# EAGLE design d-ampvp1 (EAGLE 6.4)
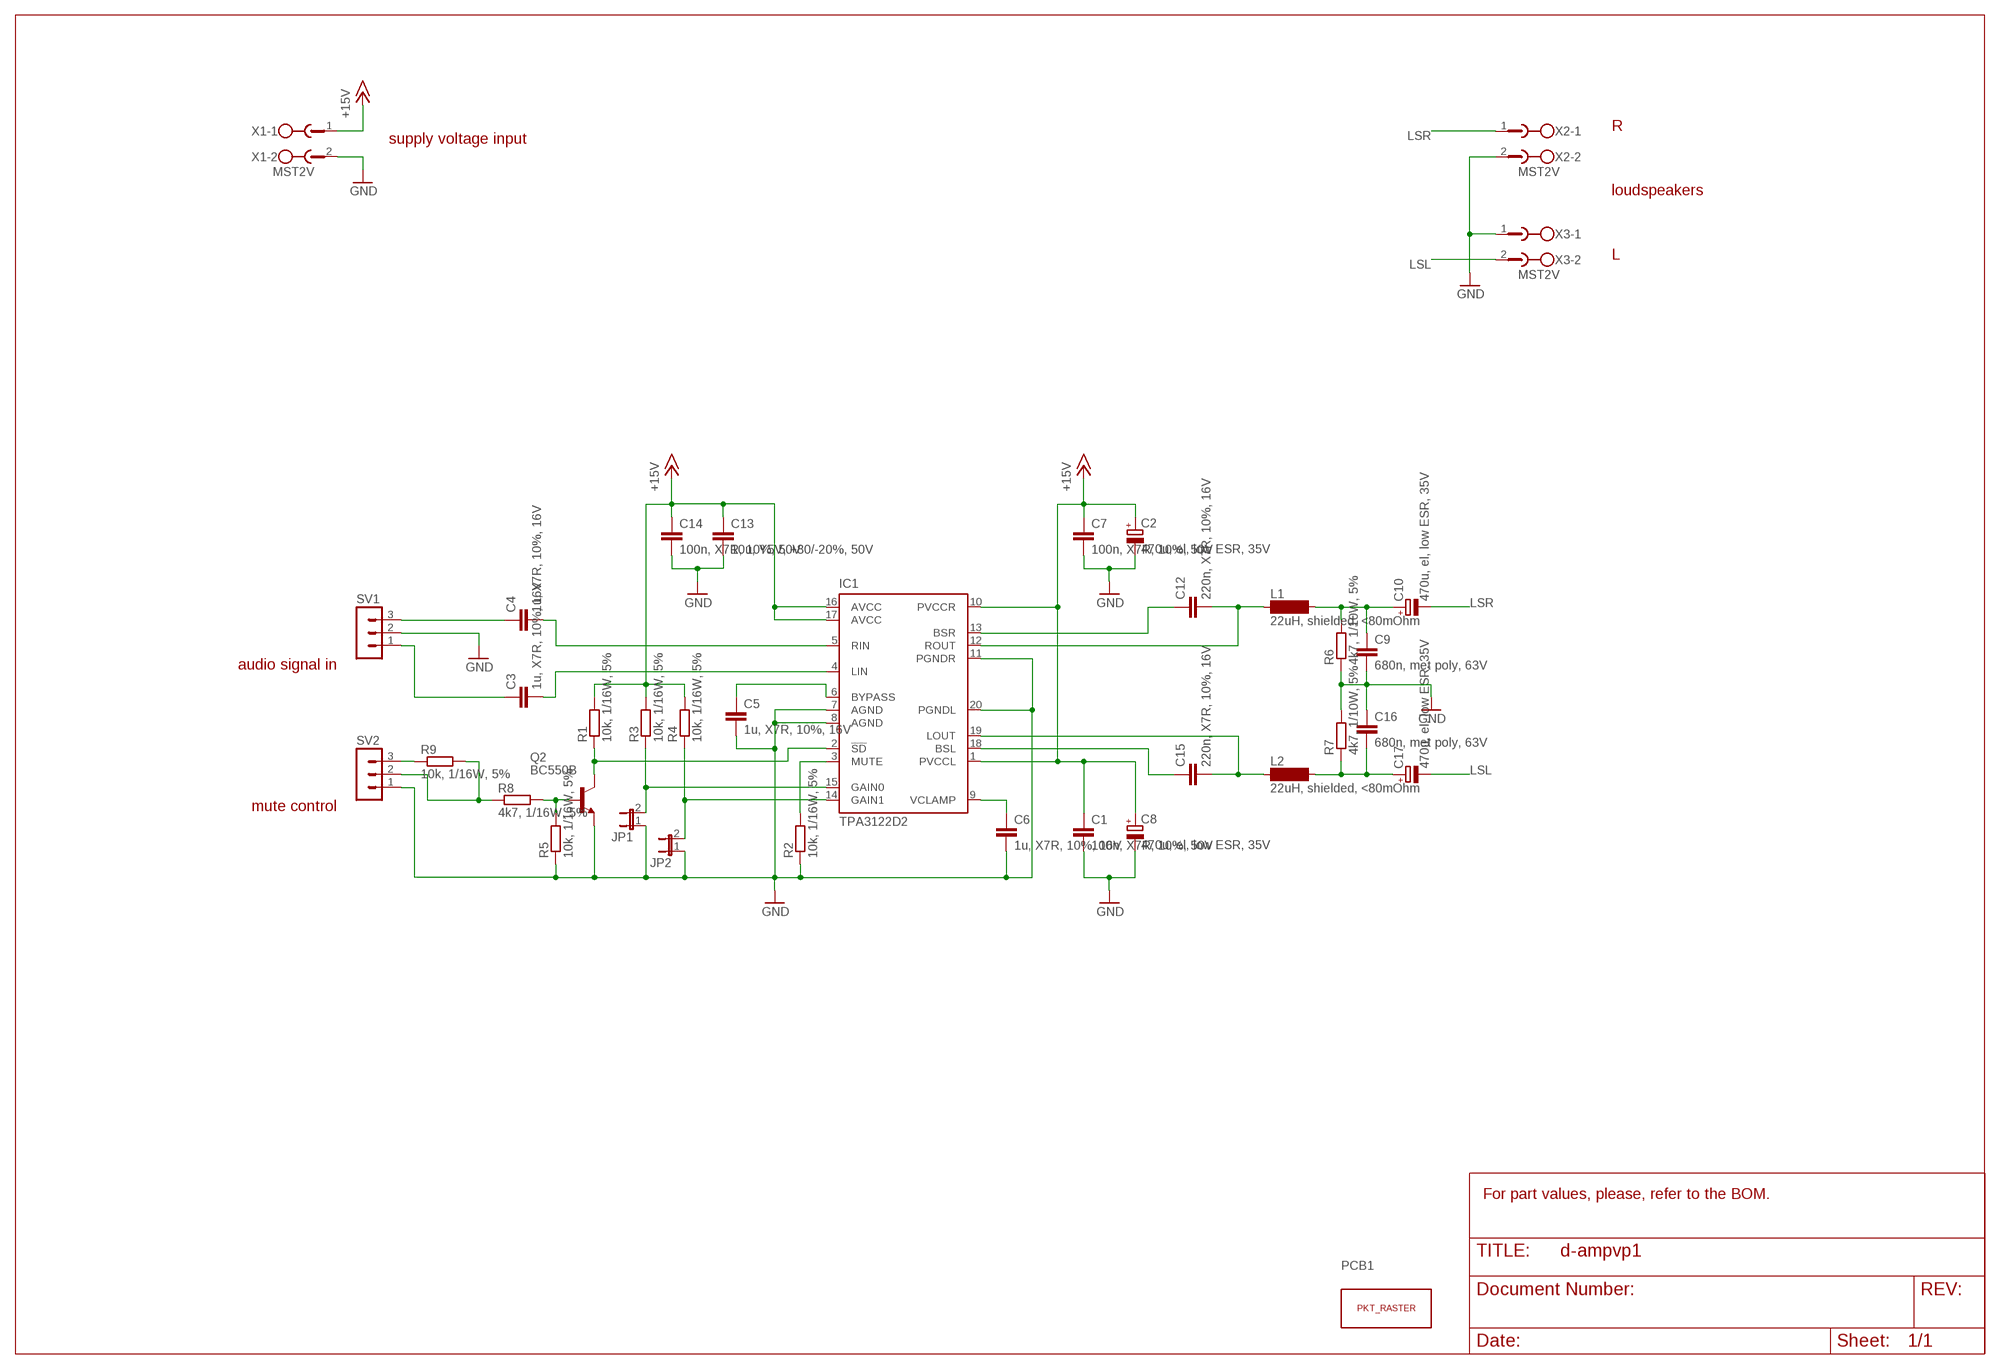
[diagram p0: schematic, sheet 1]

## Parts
C1  100n, X7R, 10%, 50V  C-EU050-025X075  [C050-025X075]
C2  470u, el, low ESR, 35V  CPOL-EUE5-13  [E5-13]
C3  1u, X7R, 10%, 16V  C-EUC1210  [C1210]
C4  1u, X7R, 10%, 16V  C-EUC1210  [C1210]
C5  1u, X7R, 10%, 16V  C-EUC1210  [C1210]
C6  1u, X7R, 10%, 16V  C-EUC1210  [C1210]
C7  100n, X7R, 10%, 50V  C-EU050-025X075  [C050-025X075]
C8  470u, el, low ESR, 35V  CPOL-EUE5-13  [E5-13]
C9  680n, met poly, 63V  C-EU075-052X106  [C075-052X106]
C10  470u, el, low ESR, 35V  CPOL-EUE5-13  [E5-13]
C12  220n, X7R, 10%, 16V  C-EU050-025X075  [C050-025X075]
C13  10u, Y5V, +80/-20%, 50V  C-EUC1210  [C1210]
C14  100n, X7R, 10%, 50V  C-EU050-025X075  [C050-025X075]
C15  220n, X7R, 10%, 16V  C-EU050-025X075  [C050-025X075]
C16  680n, met poly, 63V  C-EU075-052X106  [C075-052X106]
C17  470u, el, low ESR, 35V  CPOL-EUE5-13  [E5-13]
IC1  TPA3122D2  [DIL20]
JP1  JP1E  [JP1]
JP2  JP1E  [JP1]
L1  22uH, shielded, <80mOhm  SD12K100  [SD12K100]
L2  22uH, shielded, <80mOhm  SD12K100  [SD12K100]
PCB1  PUNKTRASTER  [PUNKTRASTER]
Q2  BC550B  [TO92-EBC]
R1  10k, 1/16W, 5%  R-EU_0204/2V  [0204V]
R2  10k, 1/16W, 5%  R-EU_0207/10  [0207/10]
R3  10k, 1/16W, 5%  R-EU_0204/7  [0204/7]
R4  10k, 1/16W, 5%  R-EU_0204/7  [0204/7]
R5  10k, 1/16W, 5%  R-EU_0204/7  [0204/7]
R6  4k7, 1/10W, 5%  R-EU_0204/7  [0204/7]
R7  4k7, 1/10W, 5%  R-EU_0204/7  [0204/7]
R8  4k7, 1/16W, 5%  R-EU_0204/7  [0204/7]
R9  10k, 1/16W, 5%  R-EU_0204/7  [0204/7]
SV1  MA03-1  [MA03-1]
SV2  MA03-1  [MA03-1]
X1  MST2V  [MSTBV2]
X2  MST2V  [MSTBV2]
X3  MST2V  [MSTBV2]

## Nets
+15V: C1.1 C2.+ C7.1 C8.+ C13.1 C14.1 IC1.1(PVCCL) IC1.10(PVCCR) IC1.16(AVCC) IC1.17(AVCC) R1.2 R3.2 R4.2 X1.1
GND: C1.2 C2.- C5.2 C6.2 C7.2 C8.- C9.2 C13.2 C14.2 C16.1 IC1.7(AGND) IC1.8(AGND) IC1.11(PGNDR) IC1.20(PGNDL) JP1.1 JP2.1 Q2.E R2.1 R5.1 R6.1 R7.2 SV1.2 SV2.1 X1.2 X2.2 X3.1
LSL: C17.- X3.2
LSR: C10.- X2.1
N$1: IC1.2(!SD) Q2.C R1.1
N$2: C3.2 IC1.4(LIN)
N$3: Q2.B R5.2 R8.2
N$4: C9.1 C10.+ L1.2 R6.2
N$5: IC1.15(GAIN0) JP1.2 R3.1
N$6: IC1.14(GAIN1) JP2.2 R4.1
N$7: C16.2 C17.+ L2.2 R7.1
N$8: C6.1 IC1.9(VCLAMP)
N$9: C5.1 IC1.6(BYPASS)
N$10: C3.1 SV1.1
N$11: C4.1 SV1.3
N$12: C4.2 IC1.5(RIN)
N$13: C12.1 IC1.13(BSR)
N$14: C15.1 IC1.18(BSL)
N$15: C15.2 IC1.19(LOUT) L2.1
N$16: C12.2 IC1.12(ROUT) L1.1
N$17: R8.1 R9.2 SV2.2
N$18: R9.1 SV2.3
N$19: IC1.3(MUTE) R2.2

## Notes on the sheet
- R
- supply voltage input
- loudspeakers
- L
- audio signal in
- mute control
- For part values, please, refer to the BOM.

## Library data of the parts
C1 C3-C7 C9 C12-C16 = rcl:C-EU: CAPACITOR, European symbol
C2 C8 C10 C17 = rcl:CPOL-EU: POLARIZED CAPACITOR, European symbol
IC1 = my_conns:TPA3122D2: TPA3122D2 15W Stereo Class D Audio Power Amplifier The TPA3122D2 is a 15-W (per channel) efficient, Class-D audio power amplifier for driving stereo single ended speakers or mono bridge tied load. The TPA3122D2 can drive stereo speakers as low as 4Ω. The efficiency of the TPA3122D2 eliminates the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
JP1 JP2 = jumper:JP1E: JUMPER
L1 L2 = inductor-neosid:SD12: INDUCTOR; OC_FARNELL: unknown; OC_NEWARK: unknown
PCB1 = my_conns:PUNKTRASTER
Q2 = transistor-npn:BC550*: NPN Transistor
R1 R3-R9 = rcl:R-EU_: RESISTOR, European symbol
R2 = rcl:R-EU_: RESISTOR, European symbol; OC_REICHELT: 1/4W; PART_VALUE: 1/4W 5%
SV1 SV2 = con-lstb:MA03-1: PIN HEADER; OC_FARNELL: unknown; OC_NEWARK: unknown
X1-X3 = con-phoenix-508:MST2V: PHOENIX; OC_FARNELL: unknown; OC_NEWARK: unknown

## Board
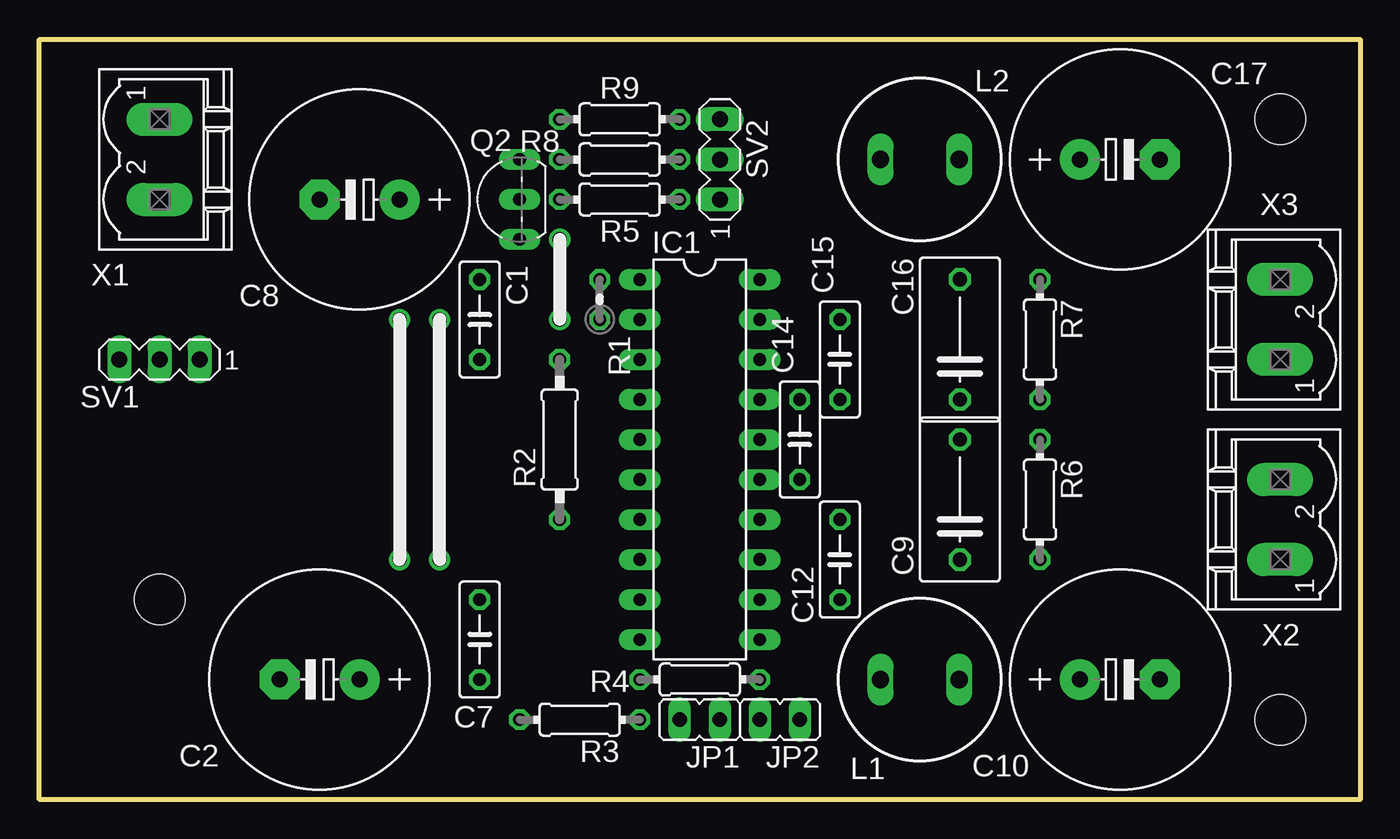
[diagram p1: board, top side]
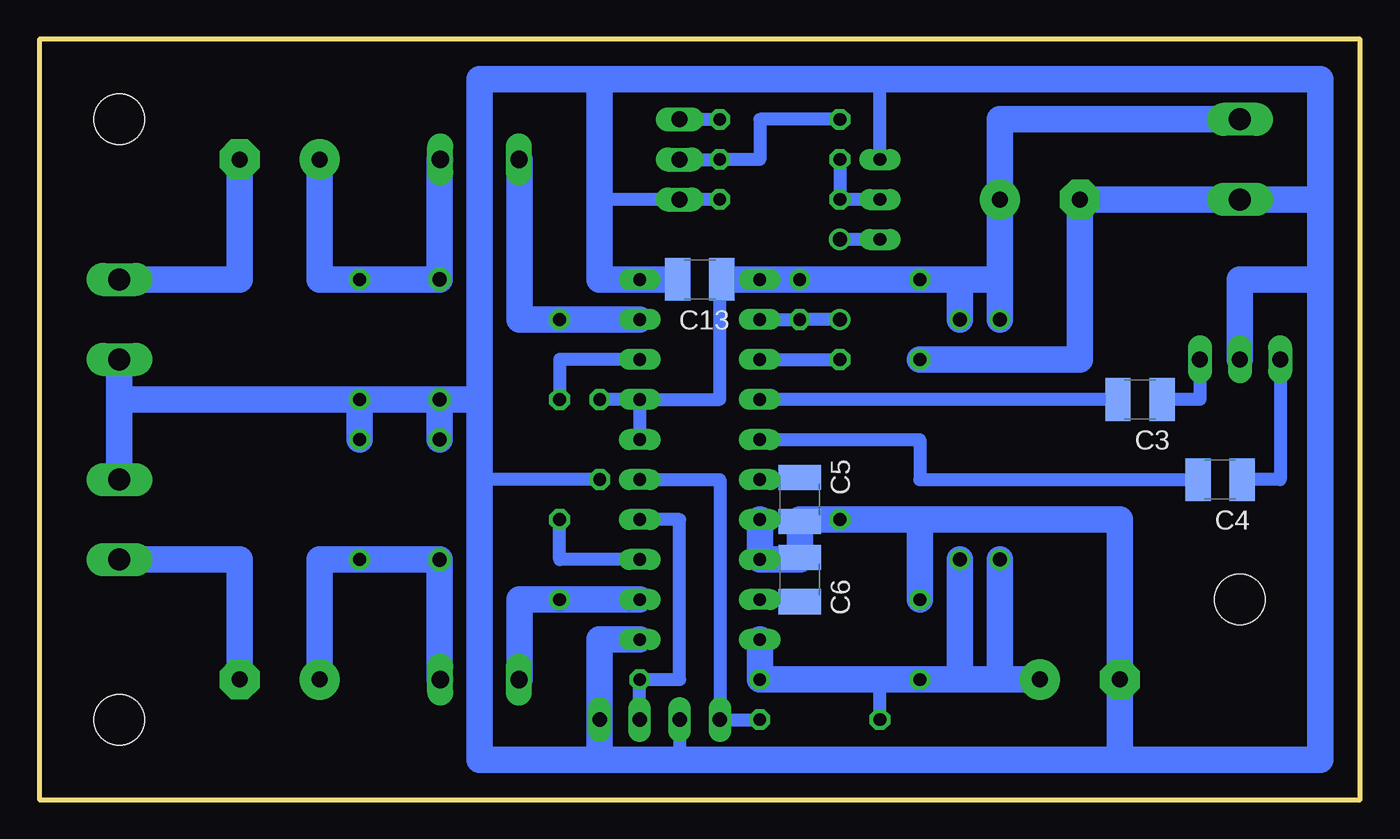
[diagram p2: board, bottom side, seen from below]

Size 83.82 x 48.26 mm. Coordinates in mm from the lower left corner, seen from the top.
Outline: 0,48.26 83.82,48.26 83.82,0 0,0 0,48.26
Copper layers (1*16): Top 0.035mm / dielectric 1.5mm / Bottom 0.035mm
Design rules "default": minimum track width 10mil, minimum drill 24mil, track to track 8mil, track to pad 8mil, pad to pad 8mil, via to via 8mil, smd to smd 8mil, copper to edge 40mil, drill to drill 8mil, minimum pad ring 10mil, minimum via ring 8mil, stop-mask expansion 4mil, vias tented up to drill 0mil, thermal gap 10mil
Holes 3.2 mm at 7.62,12.7 78.74,5.08 78.74,43.18

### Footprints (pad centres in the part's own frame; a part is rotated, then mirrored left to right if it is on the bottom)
C050-025X075 = drill 0.813 octagon: 1 -2.54,0; 2 2.54,0
E5-13 = drill 1.016 pad 2.54: + -2.54,0 | drill 1.016 pad 2.54 octagon: - 2.54,0
C1210 = smd 1.6 x 2.7: 1 -1.4,0; 2 1.4,0
C075-052X106 = drill 0.914 octagon: 1 -3.81,0; 2 3.81,0
DIL20 = drill 0.813 long: 1 -11.43,-3.81; 2 -8.89,-3.81; 3 -6.35,-3.81; 4 -3.81,-3.81; 5 -1.27,-3.81; 6 1.27,-3.81; 7 3.81,-3.81; 8 6.35,-3.81; 9 8.89,-3.81; 10 11.43,-3.81; 11 11.43,3.81; 12 8.89,3.81; 13 6.35,3.81; 14 3.81,3.81; 15 1.27,3.81; 16 -1.27,3.81; 17 -3.81,3.81; 18 -6.35,3.81; 19 -8.89,3.81; 20 -11.43,3.81
JP1 = drill 0.914 long: 1 0,-1.27; 2 0,1.27
SD12K100 = drill 1.1 long: 1 -2.5,0; 2 2.5,0
TO92-EBC = drill 0.813 long: B 0,-1.27; C -2.54,-1.27; E 2.54,-1.27
0204V = drill 0.813 octagon: 1 -1.27,0; 2 1.27,0
0207/10 = drill 0.813 octagon: 1 -5.08,0; 2 5.08,0
0204/7 = drill 0.813 octagon: 1 -3.81,0; 2 3.81,0
MA03-1 = drill 1.016 long: 1 -2.54,0; 2 0,0; 3 2.54,0
MSTBV2 = drill 1.397 long: 1 -2.54,0; 2 2.54,0

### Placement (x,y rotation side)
C1  27.94,30.48 270 top
C2  17.78,7.62 180 top
C3  13.97,25.4 180 bottom
C4  8.89,20.32 180 bottom
C5  35.56,19.05 270 bottom
C6  35.56,13.97 90 bottom
C7  27.94,10.16 90 top
C8  20.32,38.1 180 top
C9  58.42,19.05 90 top
C10  68.58,7.62 0 top
C12  50.8,15.24 270 top
C13  41.91,33.02 180 bottom
C14  48.26,22.86 270 top
C15  50.8,27.94 90 top
C16  58.42,29.21 90 top
C17  68.58,40.64 0 top
IC1  41.91,21.59 270 top
JP1  41.91,5.08 90 top
JP2  46.99,5.08 90 top
L1  55.88,7.62 0 top
L2  55.88,40.64 0 top
PCB1  2.54,2.54 0 top
Q2  29.21,38.1 90 top
R1  35.56,31.75 90 top
R2  33.02,22.86 90 top
R3  34.29,5.08 180 top
R4  41.91,7.62 180 top
R5  36.83,38.1 180 top
R6  63.5,19.05 270 top
R7  63.5,29.21 270 top
R8  36.83,40.64 180 top
R9  36.83,43.18 180 top
SV1  7.62,27.94 180 top
SV2  43.18,40.64 90 top
X1  7.62,40.64 270 top
X2  78.74,17.78 90 top
X3  78.74,30.48 90 top

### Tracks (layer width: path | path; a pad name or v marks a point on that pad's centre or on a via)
+15V  (via drill 0.9)
  Top 0.61: v25.4,30.48 v25.4,15.24 | v22.86,30.48 v22.86,15.24
  Bottom 0.813: R3.2 30.48,7.62 | IC1.17 IC1.16 | IC1.17 C14.1 | IC1.17 40.64,25.4 40.64,33.02 C13.1
  Bottom 1.676: 25.4,7.62 C7.1 30.48,7.62 R4.2 IC1.10 | 22.86,7.62 C2.+ | 22.86,33.02 C8.+ 22.86,43.18 X1.1 | v22.86,15.24 22.86,7.62 | 22.86,7.62 25.4,7.62 | 25.4,7.62 v25.4,15.24 | 22.86,33.02 25.4,33.02 | 25.4,33.02 v25.4,30.48 | 25.4,33.02 C1.1 R1.2 IC1.1 C13.1 | 22.86,33.02 v22.86,30.48
GND
  Bottom 0.813: Q2.E 30.48,45.72 | R5.1 SV2.1 48.26,38.1 | JP1.1 43.18,2.54 | C14.2 55.88,20.32
  Bottom 1.676: 2.54,38.1 2.54,33.02 | 2.54,33.02 7.62,33.02 SV1.2 | 15.24,2.54 C2.- 15.24,17.78 27.94,17.78 | 15.24,2.54 2.54,2.54 2.54,33.02 | 2.54,38.1 X1.2 C8.- 17.78,27.94 C1.2 | 2.54,38.1 2.54,45.72 30.48,45.72 48.26,45.72 | 48.26,45.72 55.88,45.72 55.88,25.4 | R7.2 C16.1 | C16.1 55.88,25.4 | 55.88,25.4 55.88,20.32 55.88,2.54 48.26,2.54 | 15.24,2.54 43.18,2.54 48.26,2.54 | C16.1 C9.2 | 48.26,45.72 48.26,38.1 48.26,33.02 IC1.20 C13.2 | C7.2 27.94,17.78 | IC1.11 48.26,10.16 JP2.1 48.26,2.54 | R7.2 78.74,25.4 X2.2 X3.1 | R7.2 R6.1 | IC1.7 IC1.8 35.56,15.24 C6.2 C5.2 35.56,17.78 R2.1 27.94,17.78
LSL
  Bottom 1.676: X3.2 71.12,33.02 C17.-
LSR
  Bottom 1.676: X2.1 71.12,15.24 C10.-
N$1  (via drill 0.9)
  Top 0.813: v33.02,35.56 v33.02,30.48
  Bottom 0.813: IC1.2 R1.1 v33.02,30.48 | Q2.C v33.02,35.56
N$2
  Bottom 0.813: C3.2 IC1.4
N$3
  Bottom 0.813: Q2.B R5.2 R8.2
N$4
  Bottom 1.676: L1.2 58.42,7.62 C9.1 R6.2 66.04,15.24 C10.+
N$5
  Bottom 0.813: R3.1 JP1.2 40.64,20.32 IC1.15
N$6
  Bottom 0.813: JP2.2 R4.1 43.18,7.62 43.18,17.78 IC1.14
N$7
  Bottom 1.676: C17.+ 66.04,33.02 R7.1 C16.2 58.42,40.64 L2.2
N$8
  Bottom 0.813: IC1.9 35.56,12.7 C6.1
N$9
  Bottom 0.813: IC1.6 35.56,20.32 C5.1
N$10
  Bottom 0.813: SV1.1 10.16,25.4 C3.1
N$11
  Bottom 0.813: SV1.3 5.08,20.32 C4.1
N$12
  Bottom 0.813: IC1.5 27.94,22.86 27.94,20.32 C4.2
N$13
  Bottom 0.813: IC1.13 50.8,15.24 C12.1
N$14
  Bottom 0.813: IC1.18 50.8,27.94 C15.1
N$15
  Bottom 1.676: IC1.19 C15.2 53.34,30.48 53.34,40.64 L2.1
N$16
  Bottom 1.676: IC1.12 C12.2 53.34,12.7 53.34,7.62 L1.1
N$17
  Bottom 0.813: SV2.2 R8.1 38.1,40.64 38.1,43.18 R9.2
N$18
  Bottom 0.813: SV2.3 R9.1
N$19
  Bottom 0.813: IC1.3 R2.2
